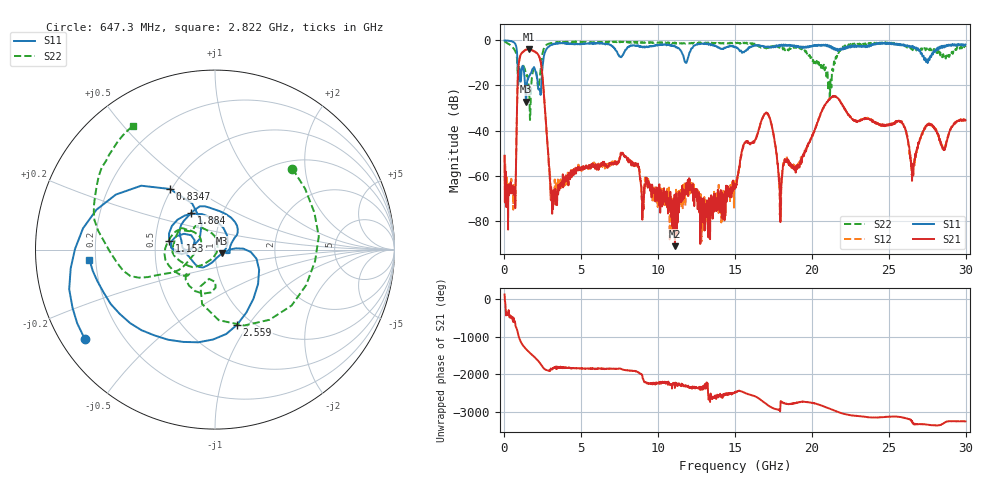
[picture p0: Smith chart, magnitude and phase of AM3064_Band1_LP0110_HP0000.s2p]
# Hz S DB R 50.0
!freq dBS11 angS11 dBS21 angS21 dBS12 angS12 dBS22 angS22
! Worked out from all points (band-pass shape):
!   1600 points, 10 MHz to 29.98 GHz, reference 50 ohm
!   highest |S21| = -3.95 dB at 1.584 GHz (marker M1); lowest = -91.3 dB at 11.09 GHz (marker M2)
!   |S21| within 3 dB of the highest: 1.025 GHz to 2.244 GHz (1.218 GHz wide, 74.5 % of centre)
!   lowest |S11| = -27.2 dB at 1.397 GHz (marker M3), VSWR 1.09, Z = 54 - j2.25 ohm
!   |S11| at or under -10 dB: 848.8 MHz to 2.507 GHz (1.659 GHz wide, 98.8 % of centre); 27.52524 GHz to 27.52801 GHz (2.776 MHz wide, 0.0101 % of centre)
!   |S22| runs from -35.3 to -0.4 dB; largest |S21 - S12| = 0.0087
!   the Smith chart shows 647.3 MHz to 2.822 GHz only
!   S11 on the Smith chart (normalised r, x): 647.3 MHz: 0.07, -0.31; 834.7 MHz: 0.49, +0.40; 1.153 GHz: 0.59, +0.06; 1.884 GHz: 0.71, +0.31; 2.559 GHz: 0.86, -0.89; 2.822 GHz: 0.18, -0.04
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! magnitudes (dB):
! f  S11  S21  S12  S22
! 10 MHz  0.0  -51.2  -51.0  -0.4
! 647.3 MHz  -1.1  -65.1  -69.0  -4.1
! 834.7 MHz  -7.5  -24.7  -24.7  -10.1
! 1.153 GHz  -11.7  -5.5  -5.4  -11.7
! 1.397 GHz  -27.2  -4.1  -4.1  -15.1
! 1.584 GHz  -16.1  -4.0  -4.0  -20.6
! 1.884 GHz  -12.2  -4.7  -4.7  -12.8
! 2.559 GHz  -7.2  -23.3  -23.3  -3.6
! 2.822 GHz  -3.1  -48.3  -47.6  -1.7
! 3.215 GHz  -1.6  -67.9  -69.5  -1.1
! 5.015 GHz  -1.4  -56.2  -57.9  -0.6
! 7.714 GHz  -6.5  -50.3  -50.3  -0.8
! 10 GHz  -2.1  -71.3  -69.9  -1.0
! 11.09 GHz  -2.6  -91.3  -76.8  -0.9
! 15 GHz  -2.9  -65.4  -62.4  -1.4
! 16.97 GHz  -2.7  -32.4  -32.3  -3.1
! 17.95 GHz  -2.3  -80.6  -79.9  -2.8
! 19.99 GHz  -2.8  -42.9  -42.7  -8.3
! 21.4 GHz  -3.4  -24.7  -24.7  -12.3
! 25 GHz  -1.1  -37.6  -37.2  -1.3
! 26.57 GHz  -2.7  -56.5  -55.9  -3.9
! 29.98 GHz  -1.9  -35.5  -34.8  -3.0
